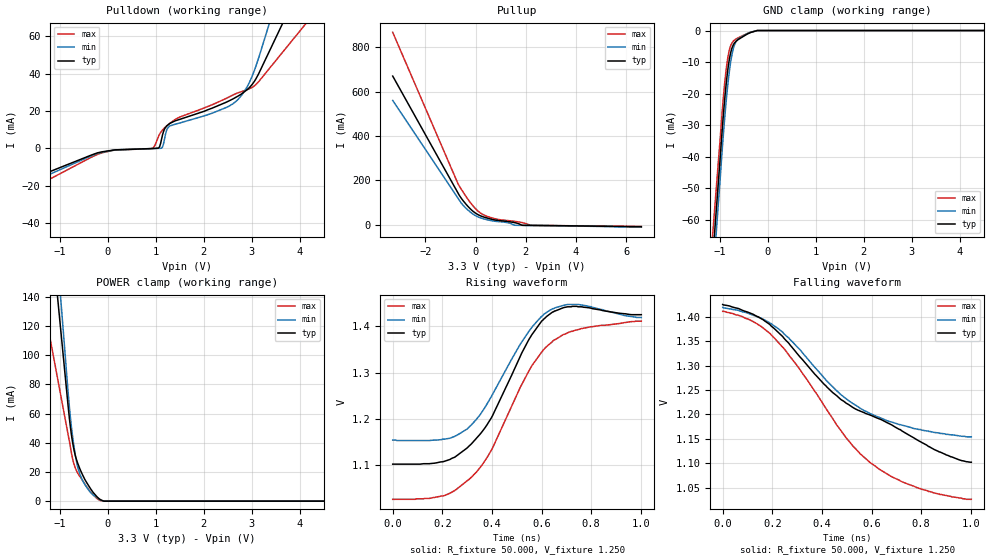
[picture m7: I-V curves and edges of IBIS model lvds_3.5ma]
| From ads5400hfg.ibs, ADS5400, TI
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[Model]   lvds_3.5ma
Model_type 3-state
Vref=1.250E+00
Rref=5.000E+01
Cref=0.000E+00
Vmeas=1.250E+00
C_comp   4.960E-13   4.830E-13   5.040E-13
[Voltage Range]   3.300E+00   3.000E+00   3.600E+00
[POWER Clamp Reference]   3.300E+00   3.000E+00   3.600E+00
[GND Clamp Reference]   0.000E+00   0.000E+00   0.000E+00
[Pullup Reference]   3.300E+00   3.000E+00   3.600E+00
[Pulldown Reference]   0.000E+00   0.000E+00   0.000E+00
[Temperature Range]   25   100   -40
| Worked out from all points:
|   slope of the pulldown table from 0 to 0.495 V, typ, clamps not added: 556 ohm
|   slope of the pullup table from 0 to 0.495 V, typ, clamps not added: 21.5 ohm
|   GND clamp passes 1 mA (typ) near -0.41 V on its own axis
|   POWER clamp passes 1 mA (typ) near -0.15 V on its own axis
|   rising waveform, R_fixture 50.000, V_fixture 1.250: 20-80 % time 186ps typ, 171ps min, 223ps max; typ from 1.1 V to 1.43 V
|   falling waveform, R_fixture 50.000, V_fixture 1.250: 20-80 % time 481ps typ, 330ps min, 342ps max; typ from 1.43 V to 1.1 V
[GND Clamp]
-3.3V     -512.5mA   -532mA     -485.3mA
-1.02V    -45.72mA   -52.47mA   -39.29mA
-940mV    -29.24mA   -35.56mA   -23.5mA
-880mV    -18.66mA   -24.35mA   -13.83mA
-840mV    -13.08mA   -18.01mA   -9.142mA
-820mV    -10.81mA   -15.22mA   -7.399mA
-760mV    -6.152mA   -8.602mA   -4.281mA
-720mV    -4.55mA    -5.747mA   -3.359mA
-660mV    -3.361mA   -3.438mA   -2.655mA
-420mV    -1.05mA    -890.2uA   -894.4uA
-220mV    0A         0A         0A
6.6V      0A         0A         0A
[Power Clamp]
-3.3V     902.6mA    1.1A       479mA
-900mV    89.47mA    104.5mA    58.13mA
-820mV    62.42mA    71.41mA    44.1mA
-760mV    45.62mA    51.12mA    33.15mA
-700mV    34.22mA    36.1mA     24.73mA
-640mV    27.04mA    25.04mA    19.92mA
-580mV    21.89mA    18.16mA    16.69mA
-480mV    14.87mA    11.41mA    11.7mA
-360mV    8.486mA    5.949mA    6.299mA
-180mV    1.609mA    1.251mA    755.8uA
-80mV     0A         0A         0A
6.6V      0A         0A         0A
[Pullup]
-3.3V     669.8mA    559.7mA    867.2mA
-700mV    142.1mA    118.7mA    184.4mA
-540mV    114.1mA    92.46mA    154.3mA
-300mV    81.32mA    64.78mA    113.2mA
-80mV     57.69mA    45.32mA    81.31mA
140mV     42.04mA    32.26mA    56.42mA
720mV     21.54mA    15.53mA    27.59mA
1.32V     12.89mA    7.434mA    17.41mA
1.56V     8.445mA    -3.27mA    14.17mA
1.88V     -3.598mA   -3.916mA   7.941mA
2.22V     -4.104mA   -4.271mA   -3.777mA
6.6V      -10.09mA   -11.93mA   -9.045mA
[Pulldown]
-3.3V     -33.82mA   -37.6mA    -44.69mA
-220mV    -2.377mA   -2.752mA   -3.215mA
940mV     -29.89uA   -56.06uA   162.1uA
1.06V     236.4uA    52.08uA    6.683mA
1.12V     5.036mA    200.4uA    9.228mA
1.18V     10.29mA    4.883mA    10.96mA
1.22V     11.8mA     9.362mA    11.92mA
1.28V     13.14mA    11.83mA    13.22mA
2.68V     27.5mA     25.36mA    29.42mA
2.94V     32.29mA    34.77mA    31.81mA
3.16V     40.83mA    49.77mA    36.24mA
6.6V      226.2mA    334.7mA    144.6mA
[Rising Waveform]
R_fixture = 50.000
V_fixture = 1.250
V_fixture_min = 1.250
V_fixture_max = 1.250
|  time   V(typ)   V(min)   V(max)
0s        1.102V     1.154V     1.026V
207.5ps   1.108V     1.156V     1.034V
257.5ps   1.12V      1.164V     1.048V
317.5ps   1.146V     1.187V     1.074V
397.5ps   1.202V     1.248V     1.132V
547.5ps   1.37V      1.388V     1.302V
600ps     1.411V     1.421V     1.344V
645ps     1.431V     1.438V     1.368V
750ps     1.442V     1.447V     1.393V
1.002ns   1.425V     1.419V     1.411V
[Falling Waveform]
R_fixture = 50.000
V_fixture = 1.250
V_fixture_min = 1.250
V_fixture_max = 1.250
|  time   V(typ)   V(min)   V(max)
0s        1.425V     1.419V     1.411V
107.5ps   1.408V     1.406V     1.394V
190ps     1.384V     1.387V     1.366V
302.5ps   1.323V     1.337V     1.298V
442.5ps   1.245V     1.257V     1.192V
525ps     1.214V     1.222V     1.135V
597.5ps   1.198V     1.201V     1.1V
792.5ps   1.145V     1.169V     1.048V
900ps     1.117V     1.159V     1.034V
1.002ns   1.102V     1.154V     1.026V
[Ramp]
dV/dt_f   1.9380E-01/5.9578E-10   1.5900E-01/3.4062E-10   2.3100E-01/3.8922E-10
dV/dt_r   1.9380E-01/1.9220E-10   1.5900E-01/1.7590E-10   2.3100E-01/2.3630E-10
R_load = 50
